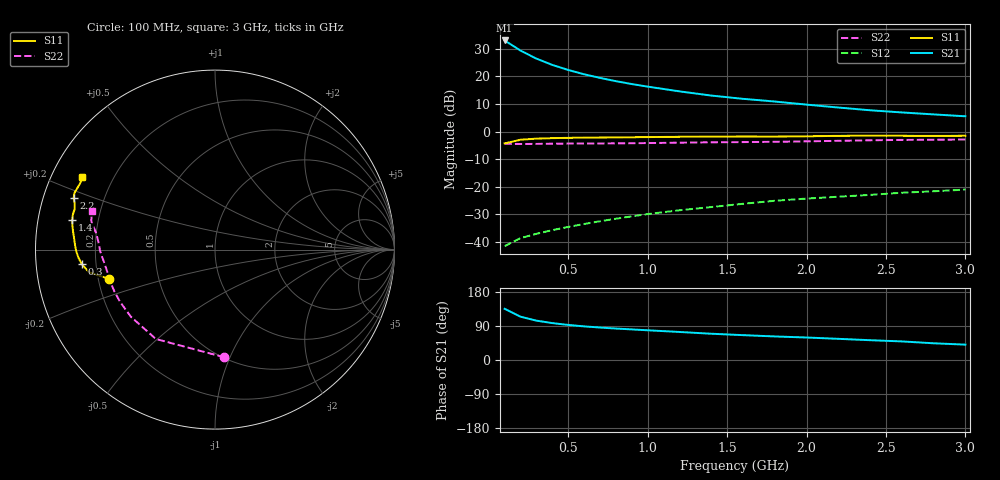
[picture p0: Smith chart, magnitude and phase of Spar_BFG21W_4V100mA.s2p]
! Filename: 4100bfg21.001
! Title: BFG21W
! Bias: Vce=4V; Ic=100mA
! Company: NXP Semiconductors NL
! User: Quality&Reliability T&D
! Measure time: 10 Nov 1999 / 11:45:44
#  MHz  S  MA  R 50
! Freq  S11  S21  S12  S22  :
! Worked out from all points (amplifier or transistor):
!   20 points, 100 MHz to 3 GHz, reference 50 ohm
!   highest |S21| = 33.1 dB at 100 MHz (marker M1)
!   |S21| within 3 dB of that: start of sweep to 181.8 MHz
!   unconditionally stable (mu >= 1): 670.6 MHz to end of sweep
!   at 400 MHz: K = 0.87, MSG = 30.0 dB, |S12| = -35.7 dB
!   at 1.2 GHz: K = 1.06, MAG = 20.0 dB, |S12| = -28.5 dB
!   at 3 GHz: K = 1.05, MAG = 11.9 dB, |S12| = -21.0 dB
!   S11 on the Smith chart (normalised r, x): 100 MHz: 0.25, -0.13; 300 MHz: 0.15, -0.05; 1.4 GHz: 0.10, +0.10; 2.2 GHz: 0.09, +0.18; 3 GHz: 0.09, +0.25
100  0.6106 -164.4  45.01 135.2  0.008377 51.6  0.6023 -85.0
200  0.7129 -169.8  29.51 114.3  0.01172 49.4  0.5971 -123.5
300  0.7469 -173.8  21.08 103.9  0.01404 52.4  0.5995 -141.3
400  0.7623 -176.7  16.22 97.4  0.01636 56.0  0.604 -151.2
500  0.7716 -178.9  13.14 92.5  0.01869 59.2  0.607 -157.5
600  0.7775 179.2  10.98 88.8  0.02114 61.7  0.6091 -161.9
700  0.7819 177.5  9.427 85.7  0.02372 64.1  0.6106 -165.3
800  0.7863 175.8  8.231 83.0  0.02634 66.1  0.6127 -168.2
900  0.7911 174.3  7.298 80.8  0.02906 67.7  0.6162 -170.7
1000  0.7965 172.9  6.551 78.4  0.032 68.7  0.6203 -172.9
1200  0.8063 170.4  5.375 74.0  0.03752 70.1  0.631 -176.5
1400  0.8123 168.3  4.511 69.3  0.04288 70.9  0.6406 -179.4
1600  0.8156 166.1  3.935 65.6  0.04912 71.4  0.646 178.0
1800  0.8139 163.7  3.516 62.1  0.05576 71.7  0.6542 175.4
2000  0.8227 161.8  3.091 59.4  0.06106 72.2  0.6665 172.5
2200  0.8389 159.8  2.737 55.9  0.06606 72.2  0.6816 170.2
2400  0.8443 158.1  2.439 52.3  0.0713 71.4  0.6973 168.5
2600  0.841 156.2  2.229 49.0  0.07799 70.4  0.7074 166.9
2800  0.8369 153.9  2.053 44.1  0.08291 68.8  0.7123 164.9
3000  0.8414 151.4  1.898 40.5  0.08888 67.8  0.7197 162.4
